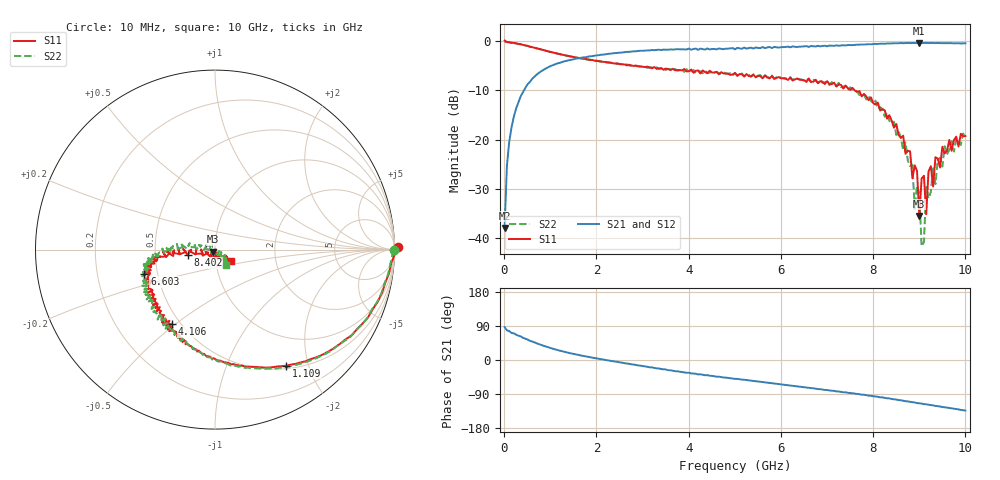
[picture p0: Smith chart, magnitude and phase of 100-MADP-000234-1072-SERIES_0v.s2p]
!Agilent Technologies,E8364C,MY48140145,A.09.42.15
!Agilent E8364C: A.09.42.15
!Date: Wednesday, December 02, 2020 08:30:15
!Correction: S11(Full 2 Port(1,2))
!S21(Full 2 Port(1,2))
!S12(Full 2 Port(1,2))
!S22(Full 2 Port(1,2))
!S2P File: Measurements: S11, S21, S12, S22:
# Hz S  dB  R 50
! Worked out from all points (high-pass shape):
!   201 points, 10 MHz to 10 GHz, reference 50 ohm
!   highest |S21| = -0.32 dB at 9.001 GHz (marker M1); lowest = -37.9 dB at 10 MHz (marker M2)
!   |S21| within 3 dB of the highest: 1.688 GHz to end of sweep
!   lowest |S11| = -35.5 dB at 9.001 GHz (marker M3), VSWR 1.03, Z = 48.8 - j1.17 ohm
!   |S11| at or under -10 dB: 7.6 GHz to end of sweep
!   |S22| runs from -41.6 to 0.0 dB; largest |S21 - S12| = 0.021
!   S11 on the Smith chart (normalised r, x): 10 MHz: -61, +51; 1.109 GHz: 0.54, -1.65; 4.106 GHz: 0.45, -0.48; 6.603 GHz: 0.42, -0.14; 8.402 GHz: 0.73, -0.04; 10 GHz: 1.18, -0.16
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1e7  0.17 0.9  -37.95 86.7  -40.98 66.2  -0.05 -0.2
5.995e7  -0.14 -4.4  -25.27 78.3  -25.17 79.3  -0.17 -4.5
2.098e8  -0.34 -14.3  -15.32 70.4  -15.30 70.1  -0.37 -14.6
1.1089e9  -2.40 -58.4  -4.67 27.9  -4.66 27.9  -2.42 -60.1
1.7083e9  -3.57 -76.9  -3.29 10.9  -3.26 11.1  -3.54 -78.7
3.35665e9  -5.51 -111.6  -1.71 -22.4  -1.70 -23.1  -5.59 -111.5
4.1059e9  -6.40 -120.3  -1.56 -35.7  -1.56 -35.5  -5.83 -124.2
5.005e9  -6.46 -133.4  -1.64 -49.8  -1.59 -49.2  -6.43 -142.5
6.6034e9  -7.61 -160.9  -1.14 -73.1  -1.16 -73.6  -7.56 -164.3
6.7033e9  -8.22 -162.9  -1.01 -75.0  -0.99 -74.6  -7.83 -167.6
8.35165e9  -15.02 178.8  -0.44 -101.4  -0.45 -102.2  -16.17 178.1
8.4016e9  -16.16 -169.3  -0.44 -102.9  -0.39 -102.4  -16.76 165.8
8.85115e9  -27.87 -155.9  -0.34 -111.4  -0.34 -111.1  -25.07 176.6
8.9011e9  -25.22 -166.9  -0.34 -112.1  -0.32 -112.6  -34.07 -176.0
8.95105e9  -26.33 -122.7  -0.37 -113.7  -0.31 -113.1  -29.31 144.5
9.001e9  -35.53 -134.5  -0.32 -114.2  -0.35 -114.1  -31.14 -143.0
9.05095e9  -27.89 -131.0  -0.36 -115.0  -0.32 -115.1  -41.64 -0.7
9.1009e9  -27.34 -76.5  -0.34 -116.5  -0.32 -115.7  -40.87 -168.9
9.15085e9  -35.13 -63.0  -0.33 -116.9  -0.37 -117.3  -29.63 -62.2
9.2008e9  -26.44 -86.8  -0.37 -118.0  -0.32 -117.9  -31.95 0.7
9.3007e9  -29.51 -51.7  -0.33 -119.7  -0.34 -120.2  -25.44 -37.0
1e10  -19.27 -37.2  -0.42 -133.4  -0.42 -133.5  -19.64 -53.1
